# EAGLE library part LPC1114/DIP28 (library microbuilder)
LPC1114 MCU DIP28 Package ARM Cortex M0, 50MHz Operation, 6 Channel 10-Bit ADC, 1²C, SPI, UART, 2x16 Bit and 2x32 Bit Timers, Internal 12MHz Oscillator, 1.8-3.6V operation.
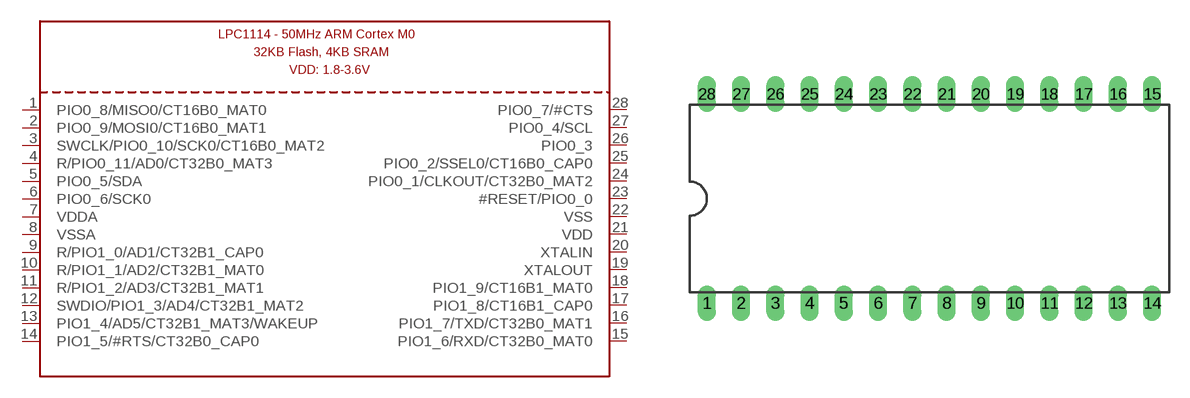
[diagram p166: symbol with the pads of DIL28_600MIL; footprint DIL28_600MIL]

Designator prefix U

## LPC1114/DIP28  [DIL28_600MIL]
1  PIO0_8/MISO0/CT16B0_MAT0
2  PIO0_9/MOSI0/CT16B0_MAT1
3  SWCLK/PIO0_10/SCK0/CT16B0_MAT2
4  R/PIO0_11/AD0/CT32B0_MAT3
5  PIO0_5/SDA
6  PIO0_6/SCK0
7  VDDA
8  VSSA
9  R/PIO1_0/AD1/CT32B1_CAP0
10  R/PIO1_1/AD2/CT32B1_MAT0
11  R/PIO1_2/AD3/CT32B1_MAT1
12  SWDIO/PIO1_3/AD4/CT32B1_MAT2
13  PIO1_4/AD5/CT32B1_MAT3/WAKEUP
14  PIO1_5/#RTS/CT32B0_CAP0
15  PIO1_6/RXD/CT32B0_MAT0
16  PIO1_7/TXD/CT32B0_MAT1
17  PIO1_8/CT16B1_CAP0
18  PIO1_9/CT16B1_MAT0
19  XTALOUT
20  XTALIN
21  VDD
22  VSS
23  #RESET/PIO0_0
24  PIO0_1/CLKOUT/CT32B0_MAT2
25  PIO0_2/SSEL0/CT16B0_CAP0
26  PIO0_3
27  PIO0_4/SCL
28  PIO0_7/#CTS

## Footprint DIL28_600MIL (pad centres in mm)
28-Pin Dual In Line (600 mil)
drill 0.813 long: 1 -16.51,-7.75; 2 -13.97,-7.75; 3 -11.43,-7.75; 4 -8.89,-7.75; 5 -6.35,-7.75; 6 -3.81,-7.75; 7 -1.27,-7.75; 8 1.27,-7.75; 9 3.81,-7.75; 10 6.35,-7.75; 11 8.89,-7.75; 12 11.43,-7.75; 13 13.97,-7.75; 14 16.51,-7.75; 15 16.51,7.75; 16 13.97,7.75; 17 11.43,7.75; 18 8.89,7.75; 19 6.35,7.75; 20 3.81,7.75; 21 1.27,7.75; 22 -1.27,7.75; 23 -3.81,7.75; 24 -6.35,7.75; 25 -8.89,7.75; 26 -11.43,7.75; 27 -13.97,7.75; 28 -16.51,7.75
